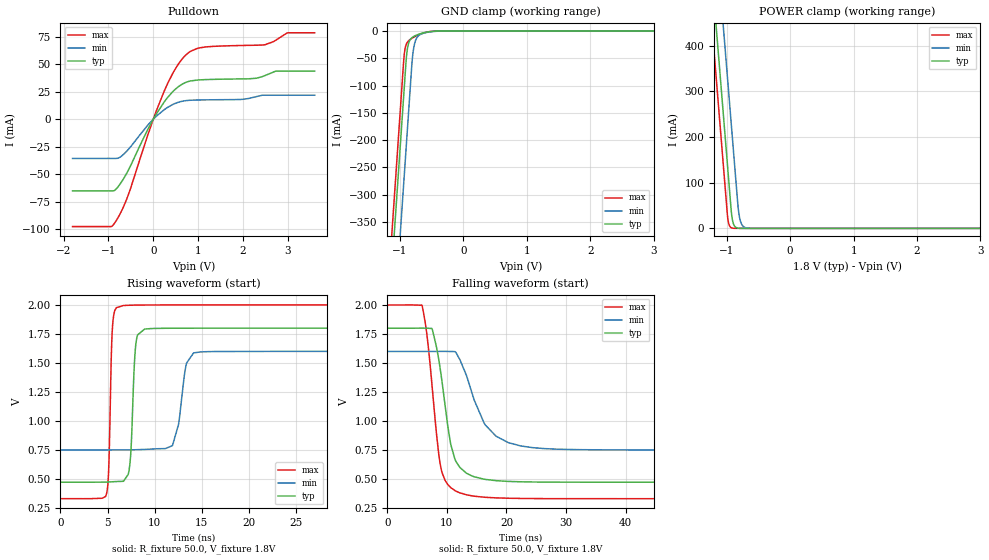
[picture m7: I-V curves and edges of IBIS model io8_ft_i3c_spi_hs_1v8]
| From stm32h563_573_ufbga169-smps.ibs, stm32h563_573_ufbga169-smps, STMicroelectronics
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[Model]   io8_ft_i3c_spi_hs_1v8
Model_type I/O_open_drain
Polarity   Non-Inverting
Enable   Active-Low
| CAP_THRESHOLD on pad IOFT is "UDTCAPC" :
| Rising=20.0% of vddiom   Falling=80.0% of vddiom
| C_comp min and max val. don't necessarily correlate with the min and max pvt
| but are the smallest and greatest pad capacitance found.
| var   typ   min   max
C_comp   3.75306pF  3.69047pF  3.87697pF
|C_comp_pulldown   3.75306pF  3.69047pF  3.87697pF
Vinl = 800.0mV
Vinh = 1.0V
Vmeas = 900.0mV   | Reference voltage for timing measurements
Cref  = 50.0pF   | Timing specification test load capacitance value
Rref  = 1.0MOhm   | Timing specification test load resistance value
Vref  = 990.0mV   | Timing specification test load voltage
[Model Spec]
| TIME_THRESHOLD on pin ZII2CV11 is "CMOS" :
| Rising=40.0% of vdd   Falling=60.0% of vdd
Vinl 703.80000mV 631.80000mV 784.80000mV
Vinh 1.06220V 937.20000mV 1.16620V
| variable   typ   min   max
[Temperature Range] 25.0 125.0 -40.0
| variable   typ   min   max
[Voltage Range] 1.8V 1.6V 2.0V
| variable   typ   min   max
[POWER Clamp Reference] 1.8V 1.6V 2.0V
| variable   typ   min   max
[GND Clamp Reference] 0V 0V 0V
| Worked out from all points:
|   slope of the pulldown table from 0 to 0.27 V, typ, clamps not added: 15.8 ohm
|   GND clamp passes 1 mA (typ) near -0.52 V on its own axis
|   POWER clamp passes 1 mA (typ) near -0.84 V on its own axis
|   rising waveform, R_fixture 50.0, V_fixture 1.8V: 20-80 % time 402ps typ, 862ps min, 285ps max; typ from 0.474 V to 1.8 V
|   falling waveform, R_fixture 50.0, V_fixture 1.8V: 20-80 % time 2.36ns typ, 4.31ns min, 1.95ns max; typ from 1.8 V to 0.474 V
[POWER Clamp]
-1.8V     1.518A     1.709A     1.407A
-1.23V    548.8mA    740.2mA    437.5mA
-1.16V    429.8mA    621.2mA    318.5mA
-1.05V    242.8mA    434.2mA    131.5mA
-980mV    123.8mA    315.2mA    17.95mA
-930mV    38.81mA    230.2mA    1.49mA
-910mV    17.82mA    196.2mA    550.8uA
-890mV    8.18mA     162.2mA    203.5uA
-810mV    363.5uA    33.6mA     3.797uA
-770mV    76.62uA    10.47mA    518.8nA
-710mV    7.416uA    1.822mA    26.34nA
3.6V      0A         0A         0A
[GND Clamp]
-1.8V     -1.579A    -1.74A     -1.515A
-1.24V    -627.3mA   -788.3mA   -562.7mA
-1.05V    -304.3mA   -465.3mA   -239.7mA
-940mV    -117.3mA   -278.3mA   -52.69mA
-930mV    -100.3mA   -261.3mA   -40.52mA
-900mV    -50.11mA   -210.3mA   -24.23mA
-880mV    -30.95mA   -176.3mA   -20.02mA
-810mV    -12.18mA   -57.97mA   -13.23mA
-780mV    -9.807mA   -29.1mA    -11.19mA
-690mV    -5.41mA    -7.142mA   -6.184mA
-420mV    -170.4uA   -446.1uA   -81.94uA
3.6V      5.755nA    953.4nA    228.2pA
| variable   typ   min   max
[Pullup Reference] 1.8V 1.6V 2.0V
| variable   typ   min   max
[Pulldown Reference] 0V 0V 0V
[Pulldown]
-1.8V     -65.02mA   -35.56mA   -97.42mA
-940mV    -65.02mA   -35.56mA   -97.42mA
-850mV    -64.17mA   -35.56mA   -93.49mA
-570mV    -47.32mA   -28.01mA   -70.04mA
-120mV    -9.088mA   -5.279mA   -14.07mA
250mV     16.04mA    8.832mA    26.05mA
520mV     28.19mA    14.82mA    47.53mA
780mV     34.17mA    17.07mA    60.14mA
1.18V     35.97mA    17.56mA    65.65mA
2.49V     39.57mA    21.77mA    67.55mA
2.99V     43.62mA    21.77mA    78.38mA
3.6V      43.62mA    21.77mA    78.38mA
[Ramp]
dV/dt_r 795.76132mV/399.70096ps 508.93417mV/786.86735ps 1.00097V/282.83544ps
dV/dt_f 795.78721mV/2.29521ns 508.98159mV/4.12093ns 1.00099V/1.94692ns
R_load = 50.0
| Removed startup time: 0s 0s 0s  .
| Removed end time: 36.4ns.
[Rising Waveform]
R_fixture   = 50.0
V_fixture   = 1.8V
V_fixture_min = 1.6V
V_fixture_max = 2.0V
0s        473.7mV    751.7mV    331.7mV
4.9ns     475mV      751.6mV    374.9mV
5.5ns     477.2mV    751.8mV    1.772V
5.95ns    479.4mV    751.8mV    1.976V
7.25ns    558.5mV    752.2mV    1.997V
8ns       1.654V     753.2mV    1.998V
8.95ns    1.792V     755.9mV    1.999V
11.9ns    1.799V     788.3mV    2V
14.15ns   1.8V       1.587V     2V
36.4ns    1.8V       1.6V       2V
| Removed startup time: 0s 0s 0s  .
| Removed end time: 99.4ns.
[Falling Waveform]
R_fixture   = 50.0
V_fixture   = 1.8V
V_fixture_min = 1.6V
V_fixture_max = 2.0V
0s        1.8V       1.6V       2V
5.85ns    1.801V     1.6V       1.993V
6.65ns    1.8V       1.6V       1.745V
7.55ns    1.79V      1.6V       1.286V
9ns       1.41V      1.601V     598.4mV
10.65ns   799.8mV    1.6V       427.5mV
12.2ns    599.9mV    1.528V     381.7mV
16.5ns    497.6mV    963.9mV    343.6mV
22.35ns   477.3mV    786.6mV    333.8mV
99.4ns    473.7mV    751.7mV    331.7mV
